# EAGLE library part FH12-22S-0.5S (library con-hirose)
0.5mm Pitch Connectors For FPC/FFC Source: Data sheet
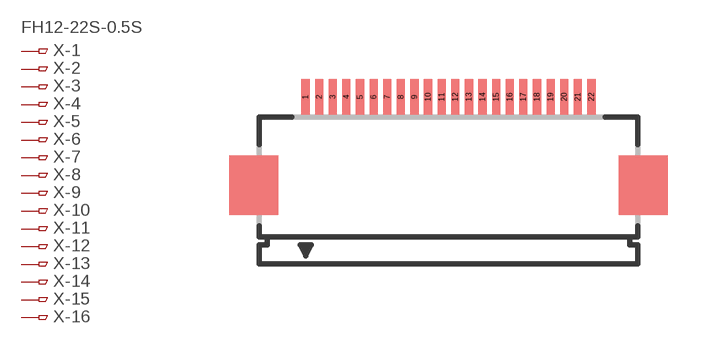
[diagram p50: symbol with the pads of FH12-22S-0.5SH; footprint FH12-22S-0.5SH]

Designator prefix X; gates -1=PINV -2=PIN -3=PIN -4=PIN -5=PIN -6=PIN -7=PIN -8=PIN -9=PIN -10=PIN -11=PIN -12=PIN -13=PIN -14=PIN -15=PIN -16=PIN -17=PIN -18=PIN -19=PIN -20=PIN -21=PIN -22=PIN

## FH12-22S-0.5SH (OC_FARNELL: 1324551; OC_NEWARK: unknown)  [FH12-22S-0.5SH]
1  -1:1  pas
2  -2:1  pas
3  -3:1  pas
4  -4:1  pas
5  -5:1  pas
6  -6:1  pas
7  -7:1  pas
8  -8:1  pas
9  -9:1  pas
10  -10:1  pas
11  -11:1  pas
12  -12:1  pas
13  -13:1  pas
14  -14:1  pas
15  -15:1  pas
16  -16:1  pas
17  -17:1  pas
18  -18:1  pas
19  -19:1  pas
20  -20:1  pas
21  -21:1  pas
22  -22:1  pas

## Footprint FH12-22S-0.5SH (pad centres in mm)
0.5mm Pitch Connectors For FPC/FFC Source: Data sheet
smd 0.3 x 1.3: 1 -5.25,3.25; 2 -4.75,3.25; 3 -4.25,3.25; 4 -3.75,3.25; 5 -3.25,3.25; 6 -2.75,3.25; 7 -2.25,3.25; 8 -1.75,3.25; 9 -1.25,3.25; 10 -0.75,3.25; 11 -0.25,3.25; 12 0.25,3.25; 13 0.75,3.25; 14 1.25,3.25; 15 1.75,3.25; 16 2.25,3.25; 17 2.75,3.25; 18 3.25,3.25; 19 3.75,3.25; 20 4.25,3.25; 21 4.75,3.25; 22 5.25,3.25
